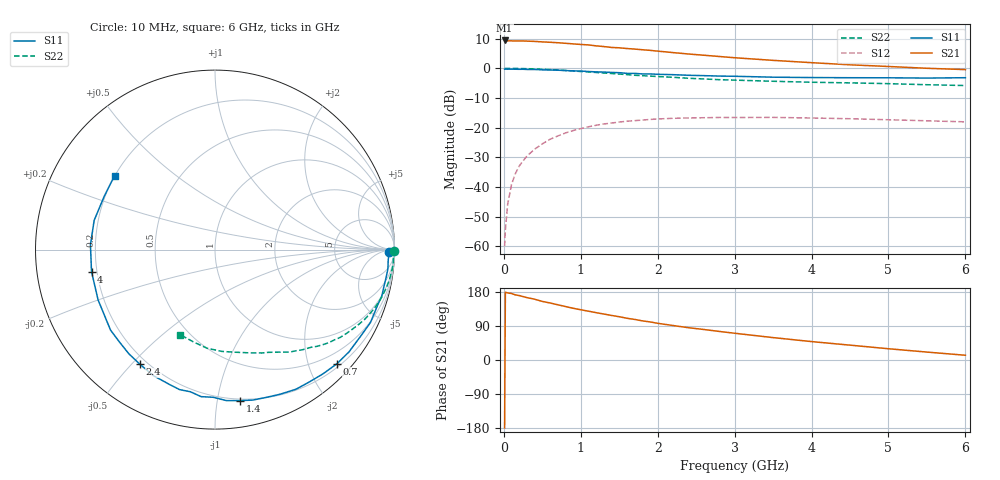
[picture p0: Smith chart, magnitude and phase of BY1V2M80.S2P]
! SIEMENS Small Signal Semiconductors
! BFY420
! Si NPN RF SIEGET Grounded Emitter Transistor in MICRO-X
! VCE = 1.25 V  IC = 0.8 mA
! Common Emitter S-Parameters:  October  1996
# GHz  S  MA  R  50
!  f  S11  S21  S12  S22
! GHz  MAG  ANG  MAG  ANG  MAG  ANG  MAG  ANG
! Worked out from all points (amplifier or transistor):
!   36 points, 10 MHz to 6 GHz, reference 50 ohm
!   highest |S21| = 9.4 dB at 10 MHz (marker M1)
!   |S21| within 3 dB of that: start of sweep to 1.742 GHz
!   unconditionally stable (mu >= 1): 4.658 GHz to end of sweep
!   at 250 MHz: K = 0.04, MSG = 20.2 dB, |S12| = -31.2 dB
!   at 1.4 GHz: K = 0.21, MSG = 12.8 dB, |S12| = -18.5 dB
!   at 6 GHz: K = 1.36, MAG = 5.2 dB, |S12| = -18.1 dB
!   S11 on the Smith chart (normalised r, x): 10 MHz: 52, -22; 700 MHz: 0.26, -2.51; 1.4 GHz: 0.19, -1.16; 2.4 GHz: 0.17, -0.53; 4 GHz: 0.18, -0.09; 6 GHz: 0.20, +0.32
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0.01  0.9679 -0.8  2.953 -179.3  0.001 99.5  0.9999 -0.3
0.02  0.97 -1.3  2.951 178.8  0.0019 89.4  0.9921 -0.6
0.05  0.9668 -3.3  2.906 177.0  0.0051 90.1  0.9969 -1.6
0.1  0.9693 -6.4  2.905 175.4  0.011 86.6  0.9951 -3.3
0.15  0.966 -9.3  2.896 171.8  0.0167 84.2  0.9952 -5.0
0.25  0.9649 -15.7  2.896 167.3  0.0275 79.6  0.9892 -8.1
0.4  0.9568 -25.1  2.848 160.4  0.0432 74.5  0.9769 -12.9
0.5  0.9437 -31.0  2.792 154.6  0.0532 70.5  0.965 -16.1
0.7  0.9308 -43.0  2.705 145.8  0.0722 63.0  0.9373 -21.9
0.9  0.9059 -54.3  2.585 136.6  0.0892 55.5  0.9027 -27.5
1.1  0.8838 -65.7  2.482 128.8  0.1032 49.0  0.8682 -32.6
1.4  0.8527 -80.6  2.25 117.6  0.1194 39.9  0.8179 -39.4
1.6  0.8228 -90.7  2.159 110.1  0.1282 34.5  0.7829 -43.5
1.8  0.8038 -99.8  2.059 103.3  0.134 29.7  0.752 -47.1
2.2  0.7817 -116.1  1.843 91.0  0.1435 20.8  0.706 -54.0
2.4  0.7637 -123.2  1.746 85.2  0.1455 17.4  0.6797 -57.2
3  0.7347 -142.4  1.509 70.6  0.148 7.9  0.6325 -65.6
3.5  0.7091 -156.7  1.363 59.1  0.1487 1.9  0.605 -71.9
4  0.6989 -169.9  1.246 48.6  0.1452 -3.2  0.5826 -78.9
4.5  0.6944 177.8  1.147 39.2  0.1412 -7.4  0.5686 -86.1
5.5  0.6849 154.3  1.002 20.9  0.1303 -12.2  0.529 -102.8
6  0.6949 143.6  0.952 12.5  0.1251 -12.5  0.5124 -112.2
